(* Logix 5000 AddOnInstructionDefinition export AMCI_3204_AOP_Home_CCW; software revision 20.03 *)

ADD_ON_INSTRUCTION AMCI_3204_AOP_Home_CCW   (* revision 1.0, vendor AMCI, ExecuteEnableInFalse *)
VAR_INPUT
   axis_status_bits : INT; {required}
   channel_number : INT; {required}
   Programmed_speed : DINT; {required}
   Acceleration : DINT; {required}
   Deceleration : DINT; {required}
END_VAR
VAR_IN_OUT
   AMCI_3204_output_data : AM:1756_3204:O:0; {required}
END_VAR
VAR_OUTPUT
   EN : BOOL; {access Read Only, visible}
   ER : BOOL; {access Read Only, visible}
END_VAR
VAR
   command_data_block : DINT[8]; {access None}
END_VAR

ROUTINE EnableInFalse   (* ladder *)
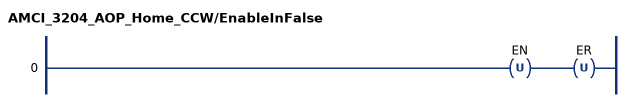
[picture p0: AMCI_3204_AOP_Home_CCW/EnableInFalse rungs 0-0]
   0: OTU(EN)OTU(ER);
END_ROUTINE

ROUTINE Logic   (* ladder *)
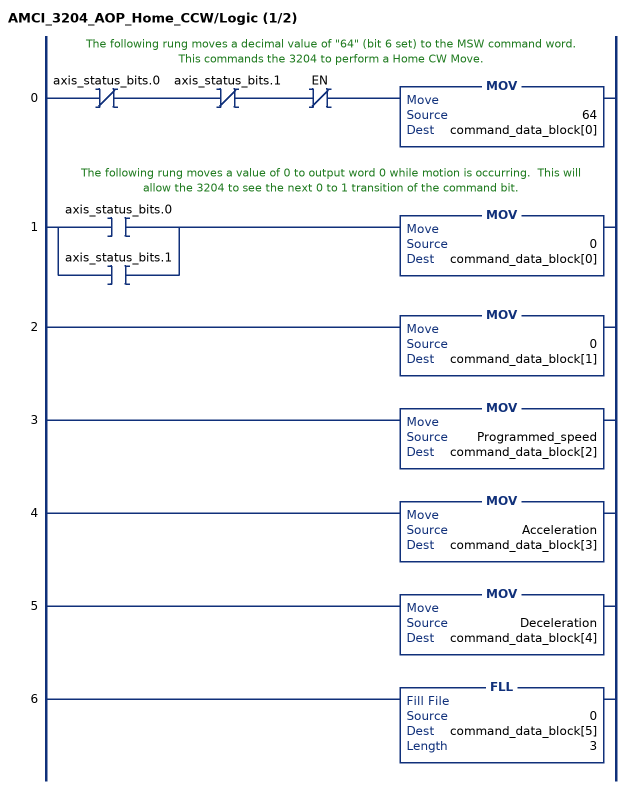
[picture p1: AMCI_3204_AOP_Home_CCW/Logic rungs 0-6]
   // The following rung moves a decimal value of "64" (bit 6 set) to the MSW command word.  This commands the 3204 to perform a Home CW Move.
   0: XIO(axis_status_bits.0)XIO(axis_status_bits.1)XIO(EN)MOV(64,command_data_block[0]);
   // The following rung moves a value of 0 to output word 0 while motion is occurring.  This will allow the 3204 to see the next 0 to 1 transition of the command bit.
   1: [XIC(axis_status_bits.0) ,XIC(axis_status_bits.1) ]MOV(0,command_data_block[0]);
   2: MOV(0,command_data_block[1]);
   3: MOV(Programmed_speed,command_data_block[2]);
   4: MOV(Acceleration,command_data_block[3]);
   5: MOV(Deceleration,command_data_block[4]);
   6: FLL(0,command_data_block[5],3);
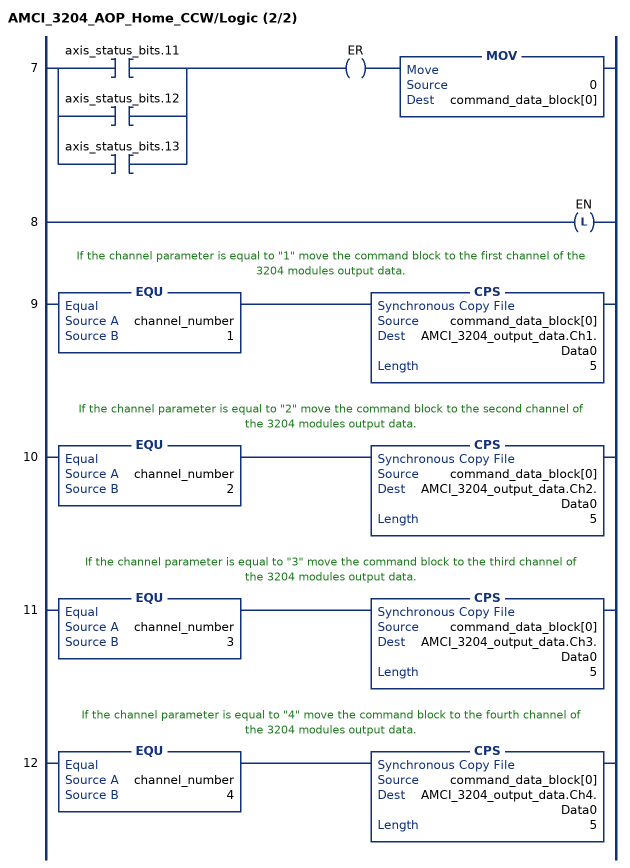
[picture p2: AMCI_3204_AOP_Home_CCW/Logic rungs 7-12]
   7: [XIC(axis_status_bits.11) ,XIC(axis_status_bits.12) ,XIC(axis_status_bits.13) ]OTE(ER)MOV(0,command_data_block[0]);
   8: OTL(EN);
   // If the channel parameter is equal to "1" move the command block to the first channel of the 3204 modules output data.
   9: EQU(channel_number,1)CPS(command_data_block[0],AMCI_3204_output_data.Ch1.Data0,5);
   // If the channel parameter is equal to "2" move the command block to the second channel of the 3204 modules output data.
   10: EQU(channel_number,2)CPS(command_data_block[0],AMCI_3204_output_data.Ch2.Data0,5);
   // If the channel parameter is equal to "3" move the command block to the third channel of the 3204 modules output data.
   11: EQU(channel_number,3)CPS(command_data_block[0],AMCI_3204_output_data.Ch3.Data0,5);
   // If the channel parameter is equal to "4" move the command block to the fourth channel of the 3204 modules output data.
   12: EQU(channel_number,4)CPS(command_data_block[0],AMCI_3204_output_data.Ch4.Data0,5);
END_ROUTINE
END_ADD_ON_INSTRUCTION
